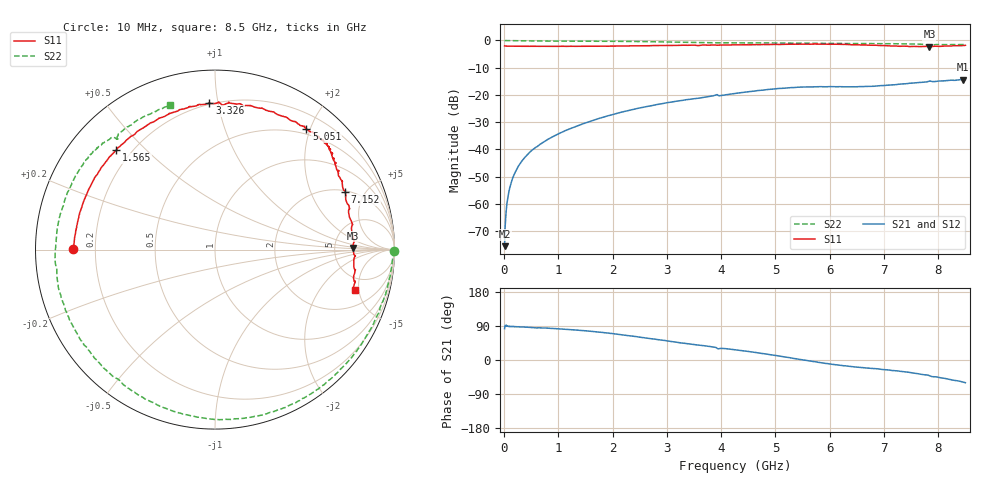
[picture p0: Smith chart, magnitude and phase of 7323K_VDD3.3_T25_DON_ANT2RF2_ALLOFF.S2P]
!Agilent Technologies,E5071C,MY46417908,A.11.23
!Date: Mon Jan 18 17:06:46 2021
!Data & Calibration Information:
!Freq	S11:SOLT2(ON)	S21:SOLT2(ON)	S12:SOLT2(ON)	S22:SOLT2(ON)
!PortZ  Port1:50+j0  Port2:50+j0
!Above PortZ is port z conversion or system Z0 setting when saving the data.
!When reading, reference impedance value at option line is always used.
# Hz S dB R 50
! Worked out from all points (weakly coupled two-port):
!   1601 points, 10 MHz to 8.5 GHz, reference 50 ohm
!   highest |S21| = -14.40 dB at 8.458 GHz (marker M1); lowest = -75.6 dB at 10 MHz (marker M2)
!   lowest |S11| = -2.3 dB at 7.837 GHz (marker M3), VSWR 7.64, Z = 381 + j17.3 ohm
!   |S11| at or under -10 dB: nowhere
!   |S22| runs from -1.8 to 0.0 dB; largest |S21 - S12| = 0.0036
!   S11 on the Smith chart (normalised r, x): 10 MHz: 0.12, +0.00; 1.565 GHz: 0.14, +0.41; 3.326 GHz: 0.19, +0.94; 5.051 GHz: 0.42, +1.94; 7.152 GHz: 2.08, +3.59; 8.5 GHz: 3.43, -4.57
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1e7  -2.05 179.7  -75.57 82.5  -74.91 83.6  -0.01 -0.4
6.30625e7  -2.08 178.1  -58.50 89.1  -58.44 89.3  -0.07 -2.4
1.055125e8  -2.09 176.9  -54.05 88.9  -54.06 88.6  -0.09 -3.7
1.851062e8  -2.11 174.6  -49.30 88.3  -49.30 88.3  -0.11 -6.2
3.0715e8  -2.15 171.1  -44.88 87.0  -44.86 87.3  -0.13 -10.2
4.875625e8  -2.15 166.0  -40.80 86.0  -40.80 86.0  -0.18 -16.1
7.210375e8  -2.16 159.4  -37.43 84.4  -37.45 84.4  -0.23 -23.2
1.426769e9  -2.13 139.1  -30.82 77.8  -30.82 77.8  -0.30 -44.7
1.564731e9  -2.15 134.9  -29.85 76.2  -29.86 76.2  -0.30 -48.9
2.312912e9  -2.02 114.1  -25.65 63.8  -25.65 63.8  -0.37 -73.0
2.843538e9  -1.90 101.7  -23.45 53.6  -23.45 53.6  -0.50 -91.7
3.326406e9  -1.75 92.2  -21.88 44.1  -21.89 44.0  -0.67 -109.0
4.255e9  -1.63 71.2  -19.49 27.2  -19.50 27.2  -0.89 -135.3
5.050938e9  -1.48 52.9  -17.66 11.0  -17.63 11.0  -0.94 -158.9
5.671769e9  -1.36 43.4  -17.06 -3.7  -16.98 -3.8  -1.05 176.0
6.329744e9  -1.50 39.6  -17.02 -16.1  -17.03 -15.5  -1.13 152.6
7.088538e9  -1.98 26.9  -16.40 -26.4  -16.47 -26.5  -1.20 141.1
7.152212e9  -2.02 23.9  -16.33 -27.8  -16.35 -27.7  -1.21 140.6
7.836719e9  -2.29 0.7  -14.95 -41.3  -14.97 -41.1  -1.70 131.3
8.048969e9  -2.17 -6.6  -14.89 -47.0  -14.93 -46.7  -1.51 126.0
8.45755e9  -1.85 -16.1  -14.40 -58.3  -14.53 -58.6  -1.49 109.6
8.5e9  -1.80 -16.1  -14.40 -59.9  -14.54 -59.8  -1.48 107.2
